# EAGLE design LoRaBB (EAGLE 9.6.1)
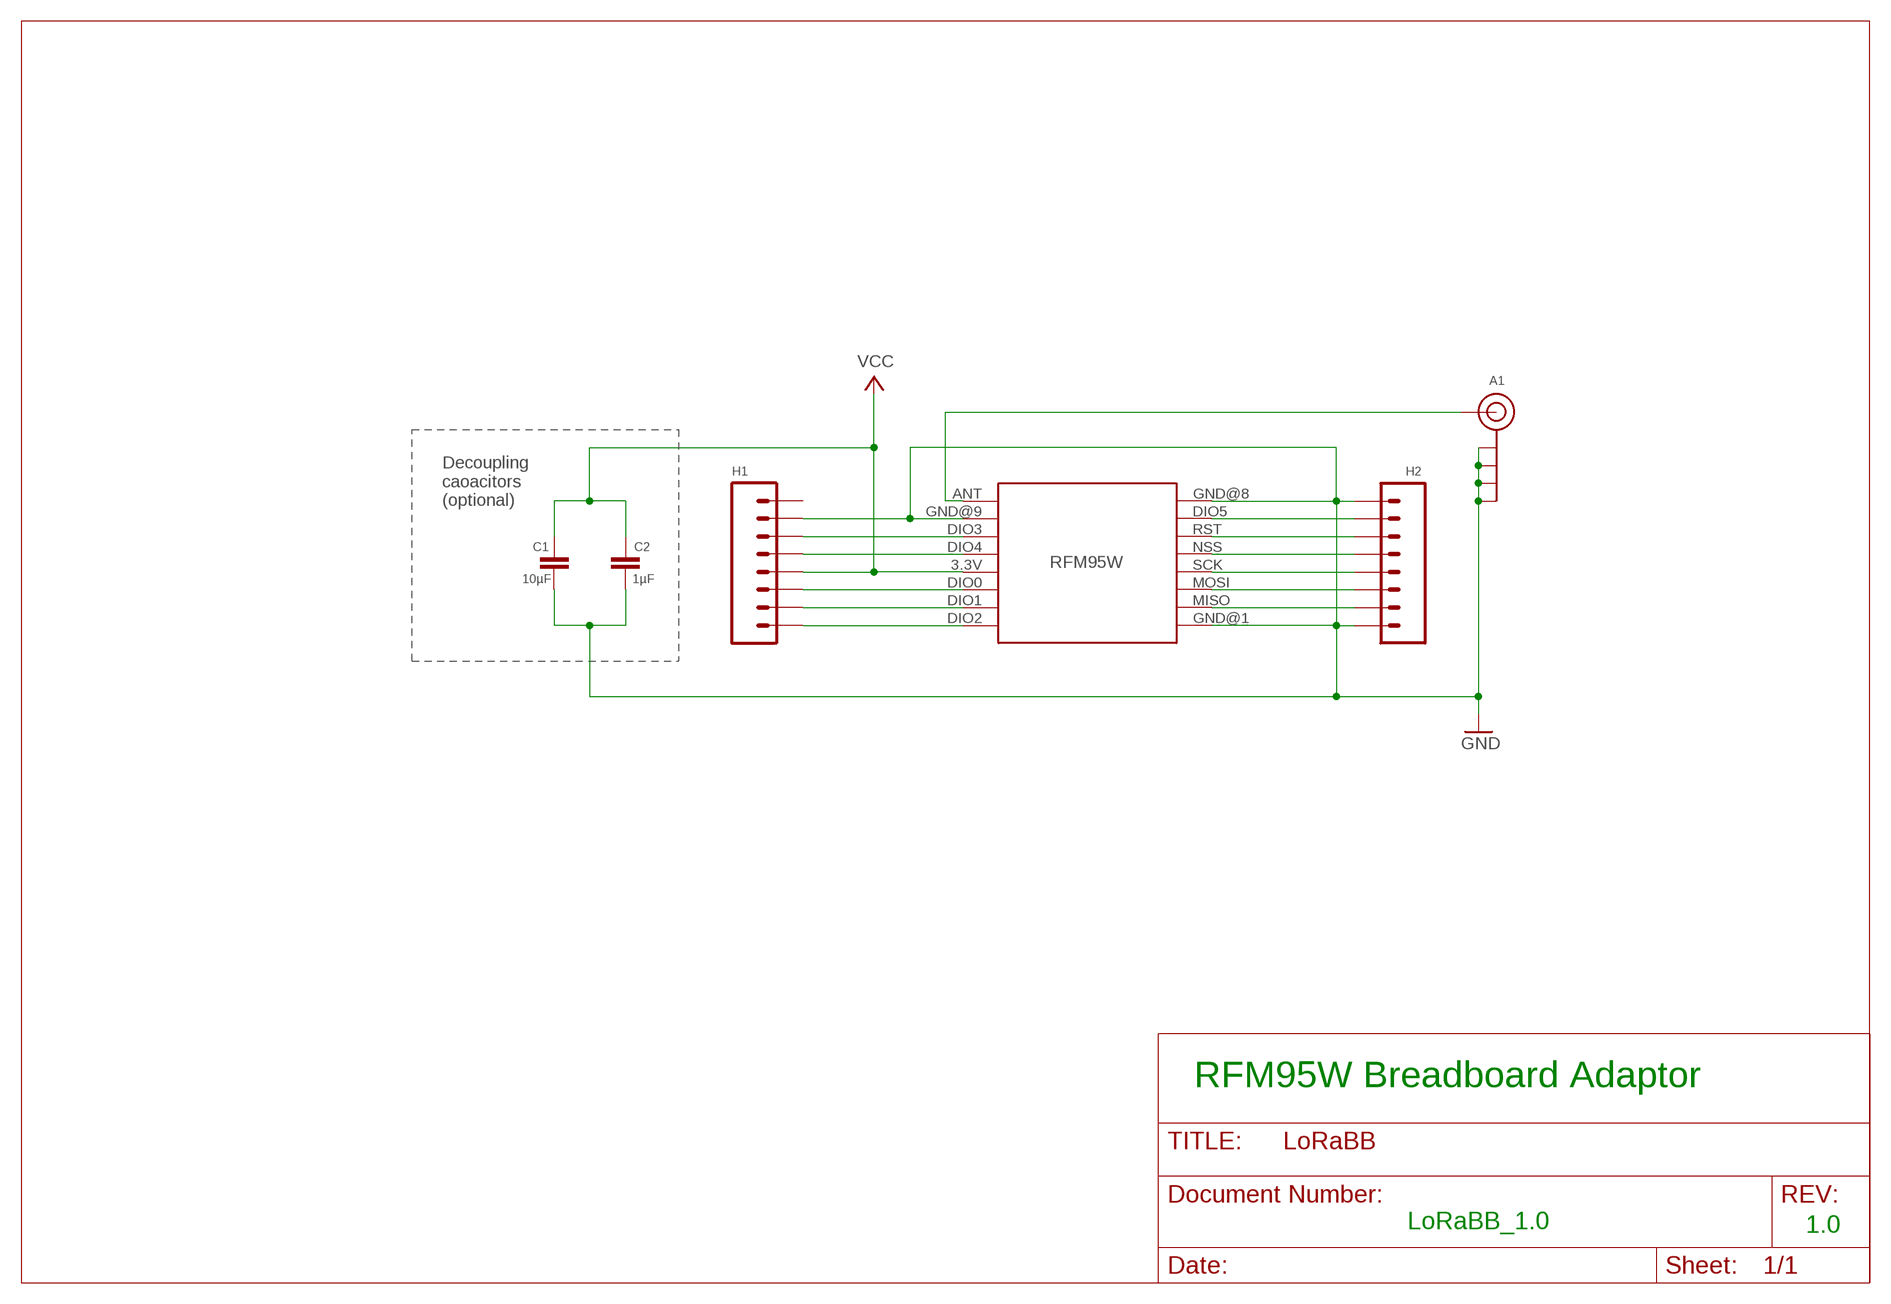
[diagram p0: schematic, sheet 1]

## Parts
A1  U.FL-SMA-EDGE-COMBO  [U.FL-SMA-EDGE-COMBO]
C1  10µF  CAPACITOR  [C0805]
C2  1µF  CAPACITOR  [C0805]
H1  1X8-PIN-HEADER  [1X8]
H2  1X8-PIN-HEADER  [1X8]
RFM95W  RFM95W-LORA  [RFM95W-LORA]

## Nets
GND: A1.GND@1A(GND) A1.GND@1B(GND) A1.GND@2A(GND) A1.GND@2B(GND) C1.2 C2.2 H1.2 H2.1 H2.8 RFM95W.GND@1(GND.1) RFM95W.GND@8(GND.2) RFM95W.GND@9(GND.3)
N$3: H2.2 RFM95W.DIO5
N$4: H2.4 RFM95W.NSS
N$8: H1.4 RFM95W.DIO4
N$9: H1.3 RFM95W.DIO3
N$11: A1.SIG RFM95W.ANT
N$12: H1.7 RFM95W.DIO1
N$13: H2.3 RFM95W.RST
N$15: H2.5 RFM95W.SCK
N$16: H2.6 RFM95W.MOSI
N$17: H2.7 RFM95W.MISO
N$27: H1.6 RFM95W.DIO0
N$32: H1.8 RFM95W.DIO2
VCC: C1.1 C2.1 H1.5 RFM95W.3.3V
Unconnected: H1.1

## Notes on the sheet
- Decoupling
  caoacitors
  (optional)
- RFM95W Breadboard Adaptor
- LoRaBB_1.0 | 1.0

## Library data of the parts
A1 = digitalconcepts:U.FL-SMA-EDGE-COMBO: Combination u.FL & SMA edge mount antenna
C1 C2 = digitalconcepts:CAPACITOR: 0805 Capacitor
H1 H2 = digitalconcepts:1X8-PIN-HEADER: Single Row 8-Pin Header
RFM95W = digitalconcepts:RFM95W-LORA: RFM95W LoRa Wireless Transceiver

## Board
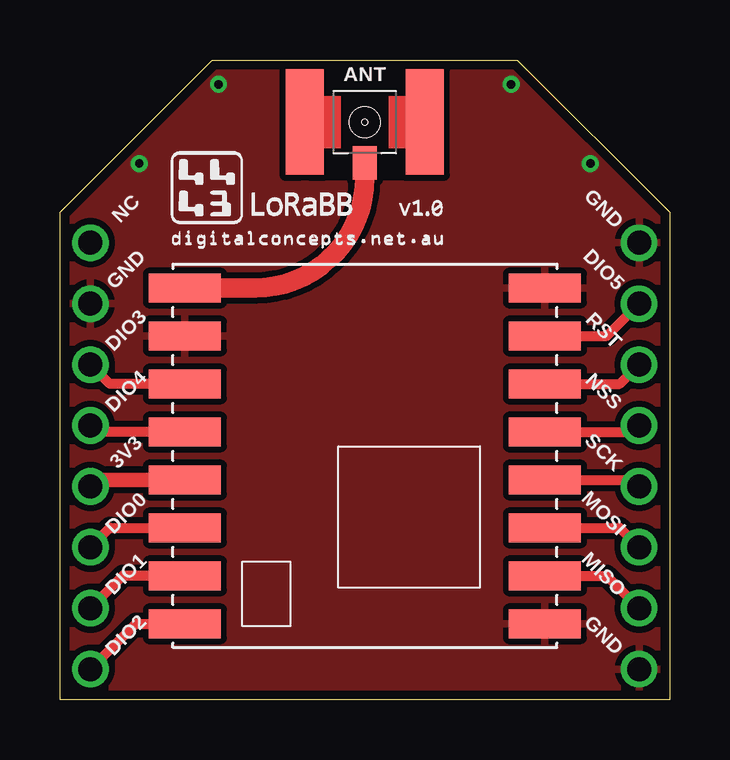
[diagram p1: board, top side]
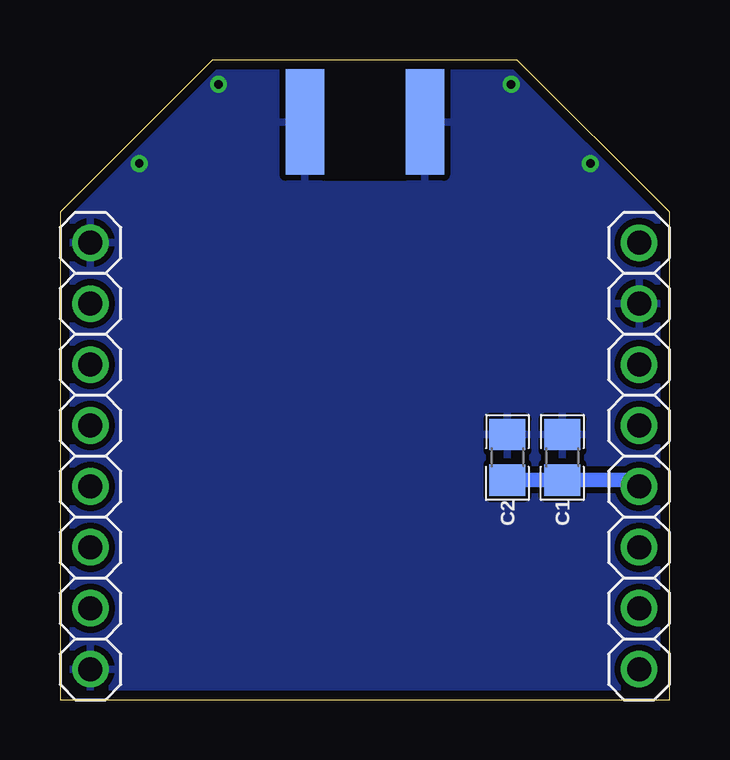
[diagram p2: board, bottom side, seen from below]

Size 25.4 x 26.67 mm. Coordinates in mm from the lower left corner, seen from the top.
Outline: 0,0 0,20.32 6.35,26.67 19.05,26.67 25.4,20.32 25.4,0 0,0
Copper layers (1*16): Top 0.0356mm / dielectric 1.5011mm / Bottom 0.0356mm
Design rules "PCBs_io": minimum track width 6mil, minimum drill 13mil, track to track 6mil, track to pad 6mil, pad to pad 6mil, via to via 6mil, smd to smd 6mil, copper to edge 15mil, drill to drill 6mil, minimum pad ring 7mil, minimum via ring 7mil, stop-mask expansion 3mil, vias tented up to drill 0mil, thermal gap 10mil

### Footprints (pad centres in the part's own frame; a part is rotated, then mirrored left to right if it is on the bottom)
U.FL-SMA-EDGE-COMBO = smd 1.6 x 4.4: GND@1A -2.5,0; GND@2A 2.5,0 | smd 1.6 x 4.4 bottom: GND@1B -2.5,0; GND@2B 2.5,0 | smd 1 x 1.4: SIG 0,-1.7
C0805 = smd 1.3 x 1.5: 1 -0.95,0; 2 0.95,0
1X8 = drill 1 pad 1.524: 1 0,0; 2 2.54,0; 3 5.08,0; 4 7.62,0; 5 10.16,0; 6 12.7,0; 7 15.24,0; 8 17.78,0
RFM95W-LORA = smd 3 x 1.2: 3.3V 7.5,1; ANT 7.5,-7; DIO0 7.5,3; DIO1 7.5,5; DIO2 7.5,7; DIO3 7.5,-3; DIO4 7.5,-1; DIO5 -7.5,-5; GND@1 -7.5,7; GND@8 -7.5,-7; GND@9 7.5,-5; MISO -7.5,5; MOSI -7.5,3; NSS -7.5,-1; RST -7.5,-3; SCK -7.5,1

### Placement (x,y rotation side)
A1  12.7,24.08 0 top
C1  4.47,10.1 90 bottom
C2  6.76,10.1 90 bottom
H1  1.27,19.05 270 top
H2  24.13,19.05 270 top
RFM95W  12.7,10.16 180 top

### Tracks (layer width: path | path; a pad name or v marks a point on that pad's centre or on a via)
GND  (via drill 0.35)
  other vias: 3.3,22.35 6.6,25.65 18.8,25.65 22.1,22.35
  pour Top (isolate 0.254): 6.35,26.67 19.05,26.67 25.4,20.32 25.4,0 21.59,0 3.81,0 0,0 0,20.32
  pour Bottom (isolate 0.254): 6.35,26.67 19.05,26.67 25.4,20.32 25.4,0 21.59,0 3.81,0 0,0 0,20.32
N$3
  Top 0.406: H2.2 22.79,15.16 RFM95W.DIO5
N$4
  Top 0.406: H2.4 23.86,11.16 RFM95W.NSS
N$8
  Top 0.406: H1.4 1.54,11.16 RFM95W.DIO4
N$9
  Top 0.406: H1.3 2.08,13.16 RFM95W.DIO3
N$11
  Top 0.813: A1.SIG 12.7,21.75 arc-90 8.11,17.16 RFM95W.ANT
N$12
  Top 0.305: RFM95W.DIO1 4.06,5.16
  Top 0.406: H1.7 2.62,5.16 4.06,5.16
N$13
  Top 0.406: H2.3 23.32,13.16 RFM95W.RST
N$15
  Top 0.406: H2.5 23.86,9.16 RFM95W.SCK
N$16
  Top 0.406: RFM95W.MOSI 23.32,7.16 H2.6
N$17
  Top 0.406: H2.7 22.78,5.16 RFM95W.MISO
N$27
  Top 0.406: H1.6 2.08,7.16 4.32,7.16 RFM95W.DIO0
N$32
  Top 0.406: H1.8 3.16,3.16 RFM95W.DIO2
VCC
  Top 0.61: H1.5 1.54,9.16 RFM95W.3.3V
  Bottom 0.61: H1.5 1.53,9.15 C1.1 C2.1

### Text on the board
tPlace: ANT | NC | GND | GND | DIO5 | DIO3 | RST | DIO4 | NSS | 3V3 | SCK | DIO0 | MOSI | DIO1 | MISO | DIO2 | GND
